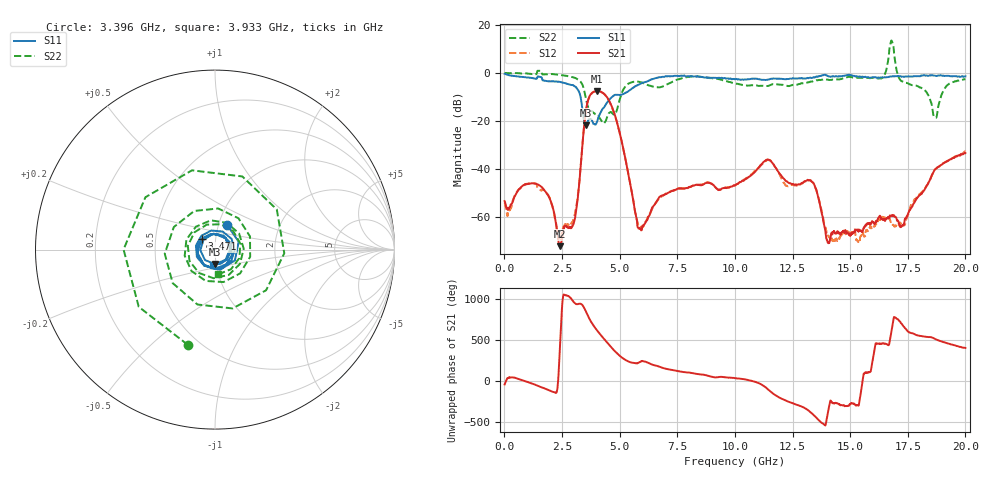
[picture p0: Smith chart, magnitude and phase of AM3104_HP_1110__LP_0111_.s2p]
!Created with skrf (http://scikit-rf.org).
# Hz S RI R 50.0
!freq ReS11 ImS11 ReS21 ImS21 ReS12 ImS12 ReS22 ImS22
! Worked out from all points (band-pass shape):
!   1601 points, 10 MHz to 20 GHz, reference 50 ohm
!   highest |S21| = -7.58 dB at 4.008 GHz (marker M1); lowest = -72.2 dB at 2.396 GHz (marker M2)
!   |S21| within 3 dB of the highest: 3.66 GHz to 4.483 GHz (822.5 MHz wide, 20.2 % of centre)
!   lowest |S11| = -21.9 dB at 3.533 GHz (marker M3), VSWR 1.18, Z = 49.5 - j8.02 ohm
!   |S11| at or under -10 dB: 3.305 GHz to 4.673 GHz (1.368 GHz wide, 34.3 % of centre)
!   |S22| runs from -21.0 to 13.5 dB; largest |S21 - S12| = 0.033
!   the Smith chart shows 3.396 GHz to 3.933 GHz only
!   S11 on the Smith chart (normalised r, x): 3.396 GHz: 1.09, +0.31; 3.471 GHz: 0.86, +0.10; 3.933 GHz: 0.97, -0.16
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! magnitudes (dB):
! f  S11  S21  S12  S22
! 10 MHz  -0.4  -53.4  -54.0  0.0
! 1.547 GHz  -1.7  -47.0  -48.6  0.8
! 2.396 GHz  -3.7  -72.2  -68.6  -0.9
! 3.021 GHz  -5.4  -62.1  -60.0  -1.9
! 3.346 GHz  -12.4  -34.8  -34.7  -4.2
! 3.396 GHz  -16.2  -28.7  -28.8  -5.2
! 3.471 GHz  -20.5  -20.9  -21.0  -7.7
! 3.533 GHz  -21.9  -16.0  -16.1  -10.4
! 3.933 GHz  -21.5  -7.7  -7.7  -17.2
! 4.008 GHz  -20.6  -7.6  -7.6  -17.7
! 4.795 GHz  -9.2  -17.6  -17.7  -17.1
! 5.857 GHz  -4.8  -64.8  -64.2  -3.8
! 6.682 GHz  -1.9  -52.4  -52.7  -6.0
! 10.01 GHz  -2.7  -46.9  -46.8  -4.4
! 11.43 GHz  -2.8  -36.0  -36.3  -5.5
! 13.34 GHz  -2.1  -45.4  -45.3  -3.6
! 14.05 GHz  -1.4  -71.0  -68.0  -2.9
! 16.36 GHz  -1.9  -60.7  -61.0  -2.3
! 16.68 GHz  -1.6  -60.6  -60.7  7.1
! 17.25 GHz  -1.5  -63.6  -63.4  -3.5
! 18.69 GHz  -1.2  -40.2  -40.2  -18.6
! 20 GHz  -1.4  -33.4  -32.7  -2.6
